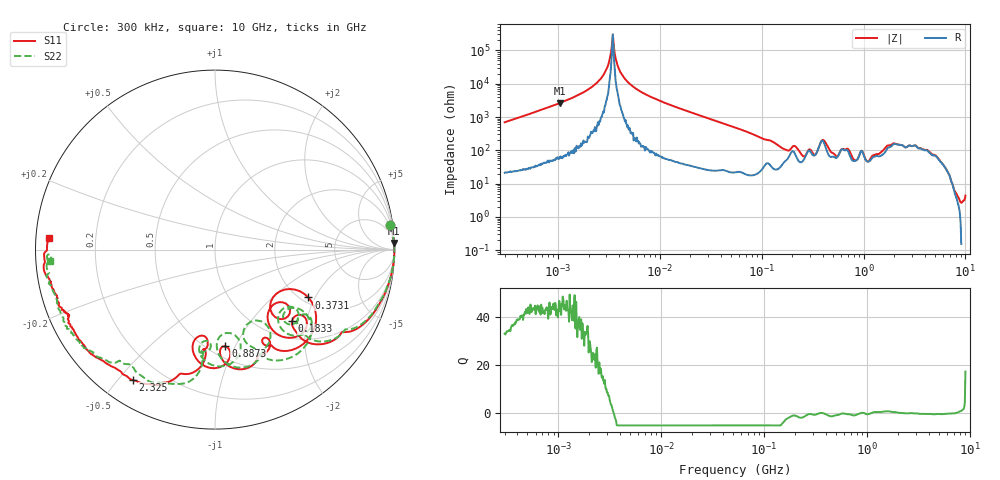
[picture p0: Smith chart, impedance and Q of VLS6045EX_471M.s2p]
! S-Parameter Data Generated by TDK Corporation
! Copyright(C) 2019 TDK Corporation.
! All Rights Reserved.
! TDK P/N: VLS6045EX-471M (Inductor)
! Property: L=470uH at 100kHz
! Size(LxWxT): 6x6x4.5mm
! Model Type: s2p (Touchstone File Format Version 1.0)
! Frequency: DC=Yes Start=0.3MHz Stop=10000MHz 802points Log-sweep
! Model Generated on May 10, 2019
! Port Assignments:
!  1 ---@@@--- 2
! Applicable Conditions:
!  Temperature = 25 degC
!  DC Bias Current = 0 A
!  Small Signal Operation
! Terms and conditions regarding TDK Simulation Models
! (1)This simulation model is being provided solely for informational purposes. Please refer to the specifications of the products in terms of detailed characteristics of such products.
! (2)In no event shall TDK Corporation of any of its subsidiaries be liable for any loss or damage arising, directly or indirectly,
!  From any information contained in this simulation model, including, but not limited to loss or damages arising from any inaccuracies, omissions or errors in connection with such information.
! (3)Any and all copyrights on this simulation model are owned by TDK Corporation.
!  Duplication or redistribution of this simulation model without prior written permission from TDK Corporation is prohibited.
! (4)This simulation model is subject to any modification or change without any prior notice.
! (5)Neither TDK Corporation nor any of its subsidiaries shall make any warranty, express or implied,
!  Including but not limited to the correctness, implied warranties of merchantability and fitness for a particular purpose with respect to this simulation models.
! (6)The use of this simulation model shall be deemed to have consented to the terms and conditions hereof.
# Hz S MA R 50
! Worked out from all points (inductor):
!   801 points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, 300 kHz to 10 GHz, reference 50 ohm
!   read as one part in series: L = 366 uH near 318.3 kHz
!   highest Q = 44.2 at 1.04 MHz (marker M1), where L = 400 uH
!   self-resonance near 3.42 MHz
!   S11 on the Smith chart (normalised r, x): 300 kHz: 2, +14; 183.3 MHz: 1.35, -1.65; 373.1 MHz: 2.18, -1.77; 887.3 MHz: 0.60, -0.92; 2.325 GHz: 0.10, -0.55; 10 GHz: 0.04, +0.04
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300000  0.9852 7.9  0.1415 -80.3  0.1416 -80.3  0.9851 7.9
1039818  0.9984 2.1  0.03816 -86.6  0.03821 -86.7  0.9984 2.1
1713600  0.9992 0.9  0.01932 -87.5  0.01927 -87.5  0.9993 0.9
2760432  0.9996 0.1  0.005794 -85.7  0.005866 -85.5  0.9995 0.1
3464350  0.9996 -0.3  0.0003326 4.5  0.000466 5.6  0.9996 -0.3
4001173  0.9995 -0.6  0.003725 83.3  0.003779 84.0  0.9997 -0.6
4673027  0.9995 -0.9  0.007792 86.2  0.007819 86.1  0.9996 -0.8
9671944  0.9987 -2.7  0.03117 86.1  0.03119 86.1  0.9989 -2.6
5.477226e7  0.9716 -16.4  0.1991 71.3  0.1991 71.3  0.9706 -15.9
1.389026e8  0.8008 -41.0  0.48 40.8  0.4801 40.8  0.8072 -39.1
1.833272e8  0.5864 -42.9  0.5357 14.2  0.5358 14.2  0.6059 -40.9
3.126428e8  0.5211 -47.6  0.5142 -4.3  0.5143 -4.3  0.5873 -45.2
3.730642e8  0.5845 -27.2  0.378 -29.0  0.3781 -29.0  0.6537 -36.4
4.508285e8  0.6938 -54.4  0.4318 0.1  0.4318 0.1  0.6947 -62.5
5.745924e8  0.5719 -59.5  0.5003 -31.4  0.5004 -31.4  0.4552 -60.1
7.235338e8  0.6851 -75.7  0.4139 -22.7  0.414 -22.7  0.6769 -75.6
8.872678e8  0.5421 -83.9  0.5148 -51.0  0.5151 -50.9  0.4687 -82.3
1.196827e9  0.491 -95.9  0.4763 -73.1  0.4772 -73.1  0.524 -92.8
1.767019e9  0.7163 -105.3  0.2123 -112.4  0.2129 -112.6  0.7781 -105.7
2.325038e9  0.8593 -122.3  0.1291 -107.4  0.1291 -108.0  0.7992 -127.0
3.816223e9  0.9078 -148.6  0.07547 -112.0  0.07459 -111.8  0.9072 -142.0
1e10  0.9276 175.9  0.05313 -151.0  0.05319 -150.9  0.92 -175.9
